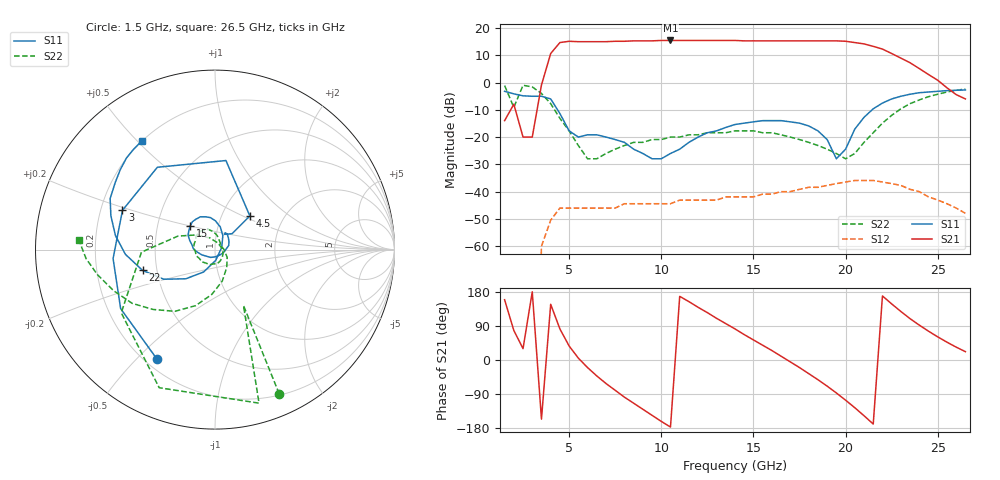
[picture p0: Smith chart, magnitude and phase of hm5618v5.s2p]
! HMMC-5618
! S-PARAMETERS  at  Vdd = 5V (single bias).  LAST UPDATED 02-07-97
#  GHZ  S  MA  R  50
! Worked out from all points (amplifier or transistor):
!   51 points, 1.5 GHz to 26.5 GHz, reference 50 ohm
!   highest |S21| = 15.4 dB at 10.5 GHz (marker M1)
!   |S21| within 3 dB of that: 4.222 GHz to 21.92 GHz (17.7 GHz wide, 135 % of centre)
!   S11 on the Smith chart (normalised r, x): 1.5 GHz: 0.25, -0.57; 3 GHz: 0.29, +0.19; 4.5 GHz: 1.35, +0.55; 15 GHz: 0.73, +0.20; 22 GHz: 0.42, -0.12; 26.5 GHz: 0.20, +0.52
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1.5  0.69 -118.0  0.2 159.0  0 -96.0  0.88 -66.0
3  0.56 157.0  0.1 180.0  0 -92.0  0.83 -112.0
3.5  0.56 125.0  0.9 -156.0  0.001 -67.0  0.63 -146.0
4  0.5 83.0  3.4 147.0  0.003 -121.0  0.41 -178.0
4.5  0.27 44.0  5.4 82.0  0.005 179.0  0.22 160.0
5  0.13 43.0  5.7 37.0  0.005 139.0  0.13 141.0
6  0.11 59.0  5.6 -20.0  0.005 94.0  0.04 65.0
7  0.1 42.0  5.6 -62.0  0.005 67.0  0.05 -27.0
8  0.08 17.0  5.7 -98.0  0.006 46.0  0.07 -66.0
10  0.04 -86.0  5.9 -162.0  0.006 12.0  0.09 -123.0
10.5  0.05 -119.0  5.9 -177.0  0.006 5.0  0.1 -137.0
12.5  0.12 178.0  5.9 125.0  0.007 -22.0  0.12 175.0
14  0.17 152.0  5.9 82.0  0.008 -40.0  0.13 144.0
15  0.19 137.0  5.8 53.0  0.008 -53.0  0.13 127.0
17  0.19 106.0  5.8 -5.0  0.01 -78.0  0.1 96.0
18.5  0.13 77.0  5.8 -52.0  0.012 -101.0  0.07 75.0
20  0.06 -86.0  5.7 -106.0  0.015 -133.0  0.04 34.0
21  0.23 -135.0  5.1 -147.0  0.016 -160.0  0.08 -32.0
22  0.42 -164.0  4.1 169.0  0.015 171.0  0.18 -77.0
22.5  0.5 -177.0  3.4 148.0  0.014 156.0  0.25 -94.0
24  0.65 154.0  1.8 92.0  0.01 118.0  0.48 -136.0
26.5  0.73 124.0  0.5 22.0  0.004 73.0  0.76 176.0
